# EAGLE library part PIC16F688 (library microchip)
14-Pin Flash-Based, 8-Bit CMOS Microcontrollers with nanoWatt Technology Source: http://ww1.microchip.com/downloads/en/DeviceDoc/41203E.pdf
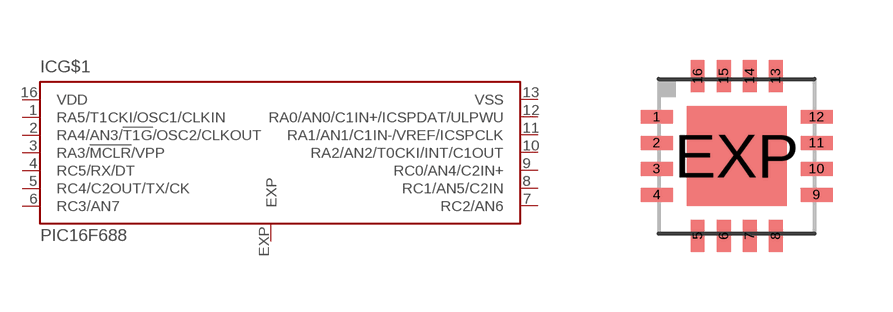
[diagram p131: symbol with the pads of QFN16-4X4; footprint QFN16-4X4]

Designator prefix IC; gates G$1=PIC16F688 EXP=EXPOSED

## PIC16F688 (MPN: PIC16F688-I/ML; OC_FARNELL: 1579588; OC_NEWARK: 56K7280)  [QFN16-4X4]
1  G$1:RA5/T1CKI/OSC1/CLKIN  in
2  G$1:RA4/AN3/!T1G!/OSC2/CLKOUT
3  G$1:RA3/!MCLR!/VPP
4  G$1:RC5/RX/DT
5  G$1:RC4/C2OUT/TX/CK
6  G$1:RC3/AN7
7  G$1:RC2/AN6
8  G$1:RC1/AN5/C2IN
9  G$1:RC0/AN4/C2IN+
10  G$1:RA2/AN2/T0CKI/INT/C1OUT
11  G$1:RA1/AN1/C1IN-/VREF/ICSPCLK
12  G$1:RA0/AN0/C1IN+/ICSPDAT/ULPWU
13  G$1:VSS  pwr
16  G$1:VDD  pwr
EXP  EXP:EXP  pas

## Footprint QFN16-4X4 (pad centres in mm)
16-Lead Plastic Quad Flat, No Lead Package (ML) - 4x4x0.9mm Body [QFN] Source: http://ww1.microchip.com/downloads/en/DeviceDoc/41203E.pdf
smd 0.8 x 0.35: 1 -2,0.975; 2 -2,0.325; 3 -2,-0.325; 4 -2,-0.975; 9 2,-0.975; 10 2,-0.325; 11 2,0.325; 12 2,0.975
smd 0.35 x 0.8: 5 -0.975,-2; 6 -0.325,-2; 7 0.325,-2; 8 0.975,-2; 13 0.975,2; 14 0.325,2; 15 -0.325,2; 16 -0.975,2
smd 2.5 x 2.5: EXP 0,0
